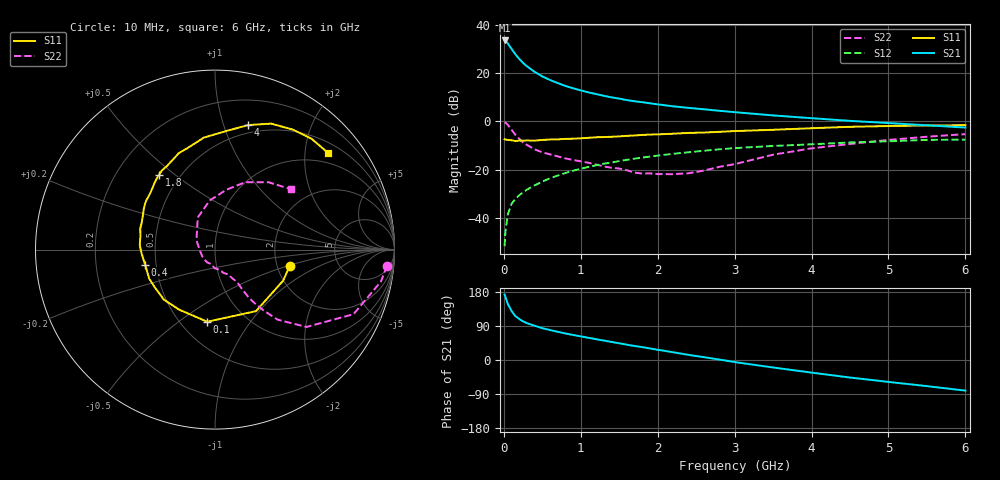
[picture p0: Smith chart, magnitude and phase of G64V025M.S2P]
! SIEMENS Small Signal Semiconductors
! BFG193
! Si NPN RF Bipolar Junction Transistor in SOT223
! VCE = 4 V  IC = 25 mA
! Common Emitter S-Parameters:  August  1996
# GHz  S  MA  R  50
!  f  S11  S21  S12  S22
! GHz  MAG  ANG  MAG  ANG  MAG  ANG  MAG  ANG
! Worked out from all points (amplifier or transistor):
!   36 points, 10 MHz to 6 GHz, reference 50 ohm
!   highest |S21| = 33.5 dB at 10 MHz (marker M1)
!   |S21| within 3 dB of that: start of sweep to 90.02 MHz
!   unconditionally stable (mu >= 1): 646.1 MHz to 2.447 GHz
!   at 250 MHz: K = 0.80, MSG = 26.8 dB, |S12| = -29.5 dB
!   at 1.4 GHz: K = 1.05, MAG = 12.1 dB, |S12| = -17.1 dB
!   at 6 GHz: K = 0.89, MSG = 2.5 dB, |S12| = -7.6 dB
!   S11 on the Smith chart (normalised r, x): 10 MHz: 2.34, -0.53; 100 MHz: 0.67, -0.64; 400 MHz: 0.43, -0.09; 1.8 GHz: 0.38, +0.44; 4 GHz: 0.42, +1.21; 6 GHz: 0.73, +2.53
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0.01  0.4259 -12.5  47.09 172.7  0.0026 89.7  0.9626 -5.4
0.02  0.4174 -24.4  45.92 166.9  0.005 80.3  0.9415 -10.9
0.05  0.412 -56.3  41.1 148.8  0.0116 73.3  0.8516 -25.0
0.1  0.4042 -96.1  31.64 129.5  0.0196 65.2  0.6678 -40.2
0.15  0.3898 -120.8  24.26 115.9  0.0248 61.0  0.5238 -48.2
0.2  0.3986 -135.8  19.55 108.2  0.0295 61.5  0.434 -51.4
0.25  0.3958 -148.0  16.13 101.9  0.0336 61.2  0.3654 -53.7
0.3  0.4008 -156.1  13.74 97.2  0.0384 62.7  0.3244 -54.9
0.4  0.3984 -167.8  10.54 90.4  0.0471 63.4  0.2633 -55.6
0.5  0.4101 -177.2  8.492 84.0  0.0564 62.8  0.2277 -55.7
0.6  0.4199 176.6  7.155 79.1  0.0663 62.8  0.2064 -56.8
0.7  0.4221 170.1  6.175 74.4  0.0753 62.4  0.1878 -58.8
0.9  0.4357 159.3  4.824 66.0  0.0951 59.2  0.1578 -61.7
1.1  0.4552 150.9  3.966 58.6  0.1134 56.6  0.1386 -69.7
1.4  0.478 139.1  3.126 47.7  0.1403 51.1  0.1092 -83.1
1.8  0.5208 126.7  2.481 33.9  0.1771 43.1  0.0829 -109.2
2.2  0.5529 115.2  2.041 20.4  0.2121 34.2  0.0805 -150.4
3.5  0.6668 83.9  1.322 -19.8  0.3087 3.8  0.2032 118.2
4  0.7184 75.0  1.159 -33.3  0.3336 -6.0  0.2754 96.1
4.5  0.7683 66.0  1.02 -46.3  0.3648 -16.1  0.3392 79.3
5.5  0.819 48.8  0.826 -69.0  0.4118 -39.4  0.4791 51.6
6  0.8292 40.5  0.742 -80.8  0.4183 -52.9  0.5422 38.3
